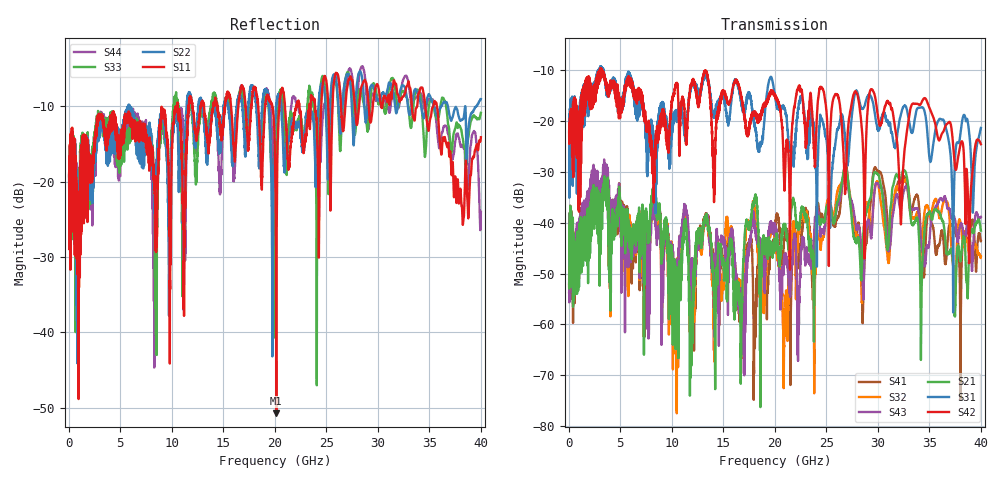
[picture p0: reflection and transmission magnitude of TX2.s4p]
!Agilent Technologies,N5245A,MY49151084,A.09.00.04
!Agilent N5245A: A.09.00.04
!Date: Thursday, January 20, 2011 08:36:44
!Correction: S11(Full 4 Port(1,2,3,4))
!S12(Full 4 Port(1,2,3,4))
!S13(Full 4 Port(1,2,3,4))
!S14(Full 4 Port(1,2,3,4))
!S21(Full 4 Port(1,2,3,4))
!S22(Full 4 Port(1,2,3,4))
!S23(Full 4 Port(1,2,3,4))
!S24(Full 4 Port(1,2,3,4))
!S31(Full 4 Port(1,2,3,4))
!S32(Full 4 Port(1,2,3,4))
!S33(Full 4 Port(1,2,3,4))
!S34(Full 4 Port(1,2,3,4))
!S41(Full 4 Port(1,2,3,4))
!S42(Full 4 Port(1,2,3,4))
!S43(Full 4 Port(1,2,3,4))
!S44(Full 4 Port(1,2,3,4))
!S4P File: Measurements: <S11,S12,S13,S14>,
!<S21,S22,S23,S24>,
!<S31,S32,S33,S34>,
!<S41,S42,S43,S44>:
# Hz S  dB  R 50
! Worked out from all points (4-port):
!   3996 points, 50 MHz to 40 GHz, reference 50 ohm
!   strongest paths, dB at 50 MHz, 10.04 GHz, 20.03 GHz, 30.02 GHz, 40 GHz:
!     S42: -22.4, -15.7, -15.2, -19.1, -24.6
!     S31: -21.9, -20.7, -15.2, -21.6, -21.4
!     S21: -52.0, -46.4, -44.7, -30.5, -41.6
!     S43: -51.1, -50.7, -41.9, -32.3, -38.9
!     S32: -52.3, -49.5, -43.4, -32.2, -46.7
!     S41: -53.7, -49.1, -42.1, -29.9, -43.6
!   lowest |S11| = -50.7 dB at 20.15 GHz (marker M1), VSWR 1.01, Z = 49.8 - j0.246 ohm
!   |S11| at or under -10 dB: start of sweep to 10.42 GHz; 20.99 GHz to 22.09 GHz (1.099 GHz wide, 5.1 % of centre); 35.73 GHz to end of sweep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
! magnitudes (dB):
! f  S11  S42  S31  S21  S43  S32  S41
! 50 MHz  -18.9  -22.4  -21.9  -52.0  -51.1  -52.3  -53.7
! 3.53 GHz  -13.8  -12.3  -12.3  -33.3  -30.1  -32.7  -30.7
! 8.44 GHz  -27.8  -24.8  -27.1  -34.0  -40.8  -37.0  -36.8
! 16.68 GHz  -7.8  -14.4  -15.3  -62.8  -53.6  -56.4  -56.8
! 18.09 GHz  -7.4  -18.7  -21.5  -34.7  -41.5  -37.9  -57.1
! 20.15 GHz  -50.7  -15.7  -16.6  -43.4  -42.0  -44.8  -39.3
! 40 GHz  -14.1  -24.6  -21.4  -41.6  -38.9  -46.7  -43.6
